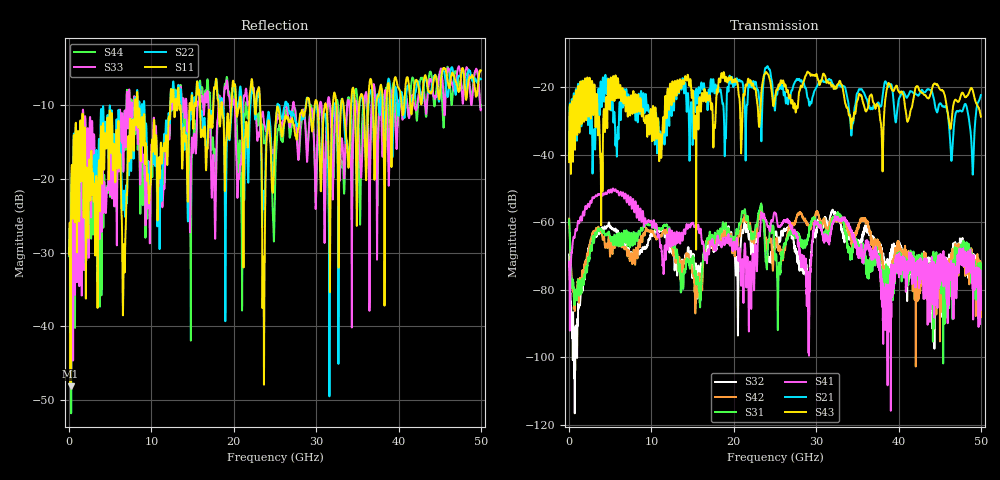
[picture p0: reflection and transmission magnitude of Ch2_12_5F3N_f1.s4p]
!Agilent Technologies,N5247A,US51170199,A.09.90.13
!Agilent N5247A: A.09.90.13
!Date: Tuesday, December 08, 2015 12:31:45
!Correction: S11(Full 4 Port(1,2,3,4))
!S12(Full 4 Port(1,2,3,4))
!S13(Full 4 Port(1,2,3,4))
!S14(Full 4 Port(1,2,3,4))
!S21(Full 4 Port(1,2,3,4))
!S22(Full 4 Port(1,2,3,4))
!S23(Full 4 Port(1,2,3,4))
!S24(Full 4 Port(1,2,3,4))
!S31(Full 4 Port(1,2,3,4))
!S32(Full 4 Port(1,2,3,4))
!S33(Full 4 Port(1,2,3,4))
!S34(Full 4 Port(1,2,3,4))
!S41(Full 4 Port(1,2,3,4))
!S42(Full 4 Port(1,2,3,4))
!S43(Full 4 Port(1,2,3,4))
!S44(Full 4 Port(1,2,3,4))
!S4P File: Measurements: <S11,S12,S13,S14>,
!<S21,S22,S23,S24>,
!<S31,S32,S33,S34>,
!<S41,S42,S43,S44>:
# Hz S  dB  R 50
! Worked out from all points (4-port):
!   3201 points, 10 MHz to 50 GHz, reference 50 ohm
!   strongest paths, dB at 10 MHz, 12.51 GHz, 25 GHz, 37.5 GHz, 50 GHz:
!     S43: -42.2, -20.0, -23.4, -25.5, -28.8
!     S21: -41.4, -21.7, -26.9, -24.6, -22.4
!     S41: -72.9, -63.3, -57.2, -70.1, -80.1
!     S31: -59.3, -64.2, -70.0, -70.3, -78.5
!     S42: -59.0, -66.3, -67.6, -65.9, -81.2
!     S32: -69.6, -69.3, -63.8, -66.8, -74.3
!   lowest |S11| = -48.1 dB at 181.8 MHz (marker M1), VSWR 1.01, Z = 50.1 - j0.385 ohm
!   |S11| at or under -10 dB: start of sweep to 7.974 GHz; 8.34 GHz to 12.29 GHz (3.947 GHz wide, 38.3 % of centre); 23.2 GHz to 28.79 GHz (5.594 GHz wide, 21.5 % of centre)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
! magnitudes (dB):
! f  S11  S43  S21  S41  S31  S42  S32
! 10 MHz  -30.2  -42.2  -41.4  -72.9  -59.3  -59.0  -69.6
! 181.8 MHz  -48.1  -29.2  -30.6  -73.6  -69.7  -69.6  -81.2
! 3.915 GHz  -13.1  -50.3  -20.6  -51.6  -62.1  -62.8  -63.3
! 5.493 GHz  -15.6  -23.4  -27.4  -50.7  -64.1  -66.6  -62.4
! 22.21 GHz  -6.6  -19.6  -20.1  -72.8  -64.9  -65.3  -68.7
! 23.65 GHz  -39.7  -16.7  -17.8  -57.7  -59.9  -58.6  -58.4
! 50 GHz  -5.4  -28.8  -22.4  -80.1  -78.5  -81.2  -74.3
